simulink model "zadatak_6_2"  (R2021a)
settings: Solver=VariableStepAuto  StartTime=0.0  StopTime=0.04  RelTol=1e-3
libraries: spsGroundLib x2, spsLoadFlowBusLib x2, spsVoltageMeasurementLib x2, spsThreePhasePISectionLineLib x1, spsThreePhaseSourceLib x1, spsThreePhaseSeriesRLCLoadLib x1, spspowerguiLib x1

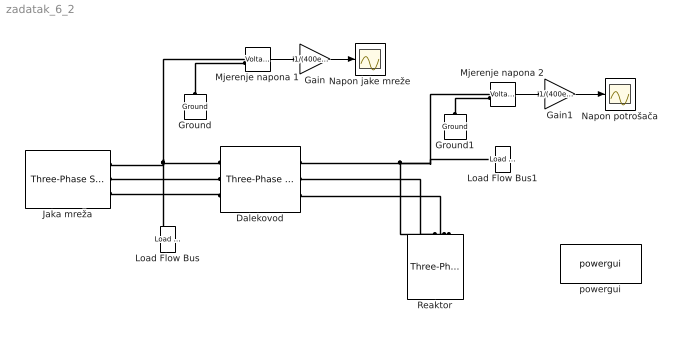
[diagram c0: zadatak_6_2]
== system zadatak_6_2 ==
  Dalekovod : spsThreePhasePISectionLineLib/Three-Phase PI Section Line  LConnTagsString=a|b|c  RConnTagsString=A|B|C  Length=100  Frequency=50  Resistances=[0.011 0.3864]  Inductances="[0.8675e-3  4.1264e-3]"  Capacitances=[13.41e-9 7.751e-9]
  Gain : Gain  Gain=1/(400e3/sqrt(3)*sqrt(2))
  Gain1 : Gain  Gain=1/(400e3/sqrt(3)*sqrt(2))
  Ground : spsGroundLib/Ground  LConnTagsString=a
  Ground1 : spsGroundLib/Ground  LConnTagsString=a
  Jaka mreža : spsThreePhaseSourceLib/Three-Phase Source  InternalConnection=Yg  VoltagePhases=off  Voltage=(400000)*1.0037  PhaseAngle=-2.6698  Voltage_phases=[25e3 25e3 25e3]/sqrt(3)  PhaseAngles_phases=[0 -120 +120]  Frequency=50  NonIdealSource=on  SpecifyImpedance=off  Resistance=180.1  Inductance=26.525e-3  ShortCircuitLevel=100e6  BaseVoltage=400e3  XRratio=7  BusType=swing  Pref=10000  Qref=0  Prefabc=[10e3, 10e3, 10e3]  Qrefabc=[0, 0, 0]  Qmin=-Inf  Qmax=Inf
  Load Flow Bus : spsLoadFlowBusLib/Load Flow Bus  LConnTagsString=a  Phases=single  Connectors=on one side  ID=1  Vbase=400e3  Vref=1  Vangle=0  VLF=1  VLFb=1  VLFc=1  angleLF=0  angleLFb=0  angleLFc=0
  Load Flow Bus1 : spsLoadFlowBusLib/Load Flow Bus  LConnTagsString=a  Phases=single  Connectors=on one side  ID=2  Vbase=400e3  Vref=1  Vangle=0  VLF=0.9872  VLFb=1  VLFc=1  angleLF=0.02602  angleLFb=0  angleLFc=0
  Mjerenje napona 1 : spsVoltageMeasurementLib/Voltage Measurement  PhasorSimulation=off  OutputType=Complex  PSBequivalent=0
  Mjerenje napona 2 : spsVoltageMeasurementLib/Voltage Measurement  PhasorSimulation=off  OutputType=Complex  PSBequivalent=0
  Napon jake mreže : Scope
  Napon potrošača : Scope
  Reaktor : spsThreePhaseSeriesRLCLoadLib/Three-Phase Series RLC Load  LConnTagsString=A|B|C  Configuration=Y (grounded)  NominalVoltage=400e3  Vabc=[1e3 1e3 1e3]  Vabcp=[1e3 1e3 1e3]  NominalFrequency=50  UnbalancedPower=off  ActivePower=366666.6667  InductivePower=110000000  CapacitivePower=0  Pabc=[10e3 9e3 11e3]  QLabc=[100 90 110]  QCabc=[100 90 110]  Pabcp=[10e3 9e3 11e3]  QLabcp=[100 90 110]  QCabcp=[100 90 110]  Measurements=None  LoadType=constant Z
  powergui : spspowerguiLib/powergui  Priority=1  SimulationMode=Continuous  SampleTime=50e-6  frequency=60  Iterations=50  frequencyindice=50  Pbase=100e6  ErrMax=1e-4  UnitsV=kV  UnitsW=MW  buscounter=0  FunctionMessages=off  echomessages=off  EnableUseOfTLC=off  CurrentSourceSwitches=off  DisableSnubberDevices=off  DisableRonSwitches=off  DisableVfSwitches=off  DisplayEquations=off  AutomaticDiscreteSolvers=off  SolverType=Tustin/Backward Euler (TBE)  Interpol=off  ExternalGateDelay=off  methode=off  Ts=100  x0status=blocks  SPID=on  SwTol=0  HookPort=off  NonlinearTolerance=1e-4  nMaxIteration=100  ContinueOnMaxIteration=off  RestoreLinks=warning  ResistiveCurrentMeasurement=off  Frange=[0:2:500]  Ylog=off  Xlog=on  ShowGrid=off  save=off  variable=ZData  structure=0  ZoomFFT=off  StartTime=0.0  cycles=1  DisplayStyle=1  fundamental=60  FreqAxis=off  MaxFrequency=1000  frequencyindicesteady=1  RmsSteady=1  display=off
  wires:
  Gain/1 -> Napon jake mreže/1
  Mjerenje napona 1/1 -> Gain/1
  Mjerenje napona 2/1 -> Gain1/1
  Gain1/1 -> Napon potrošača/1
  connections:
  Dalekovod/LConn1 -- Load Flow Bus/LConn1 -- Mjerenje napona 1/LConn1 -- Jaka mreža/RConn1
  Dalekovod/LConn2 -- Jaka mreža/RConn2
  Dalekovod/LConn3 -- Jaka mreža/RConn3
  Dalekovod/RConn1 -- Load Flow Bus1/LConn1 -- Mjerenje napona 2/LConn1 -- Reaktor/LConn1
  Dalekovod/RConn2 -- Reaktor/LConn2
  Dalekovod/RConn3 -- Reaktor/LConn3
  Ground/LConn1 -- Mjerenje napona 1/LConn2
  Ground1/LConn1 -- Mjerenje napona 2/LConn2
